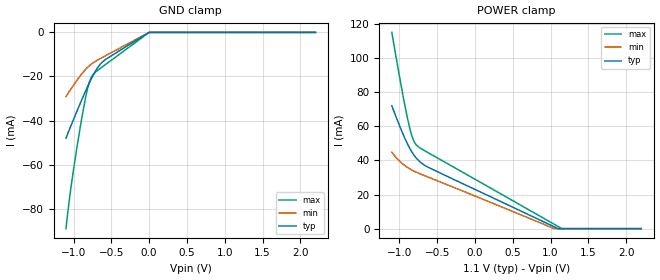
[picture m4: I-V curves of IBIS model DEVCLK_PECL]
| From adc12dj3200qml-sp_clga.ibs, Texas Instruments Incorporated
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[Model]   DEVCLK_PECL
Model_type   Input
Vinl = 0.33   | Vinl & Vinh are referred to a 1.1V supply, and are an IBIS required field.
Vinh = 0.77   | However, please note that this is a differential input.
|   typ   min   max
C_comp   1.61p   1.44p   1.78p
[Voltage Range]   1.1   1.05   1.15
[Temperature Range]   25   125   -40
[Power Clamp Reference]   1.1   1.05   1.15
[GND Clamp Reference]   0   0   0
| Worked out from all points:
|   GND clamp passes 1 mA (typ) near -0.05 V on its own axis
[GND Clamp]
|   Voltage   I(typ)   I(min)   I(max)
-1.1V     -48mA      -29.09mA   -89.09mA
-1.037V   -42.61mA   -25.83mA   -71.08mA
-997.7mV  -39.28mA   -23.83mA   -61.61mA
-911.9mV  -32.24mA   -19.74mA   -43.08mA
-845.9mV  -27.02mA   -16.98mA   -30.43mA
-816.2mV  -24.76mA   -15.92mA   -25.7mA
-779.9mV  -22.11mA   -14.81mA   -21.45mA
-753.5mV  -20.29mA   -14.12mA   -19.63mA
-684.2mV  -16.12mA   -12.62mA   -17.3mA
-581.9mV  -12.38mA   -10.7mA    -14.7mA
-1.1mV    -23.63uA   -20.45uA   -28.66uA
2.2V      0A         0A         0A
[POWER Clamp]
|   Voltage   I(typ)   I(min)   I(max)
-1.1V     71.96mA    44.84mA    115mA
-984.5mV  58.87mA    39.03mA    85.73mA
-921.8mV  52.39mA    36.79mA    70.97mA
-878.9mV  48.42mA    35.5mA     61.91mA
-842.6mV  45.49mA    34.54mA    55.55mA
-809.6mV  43.23mA    33.78mA    51.43mA
-776.6mV  41.35mA    33.09mA    49.05mA
-733.7mV  39.37mA    32.27mA    47.45mA
-647.9mV  36.58mA    30.73mA    45.22mA
1.048V    1.085mA    30.93uA    2.566mA
1.147V    0A         0A         67.28uA
2.2V      0A         0A         0A
